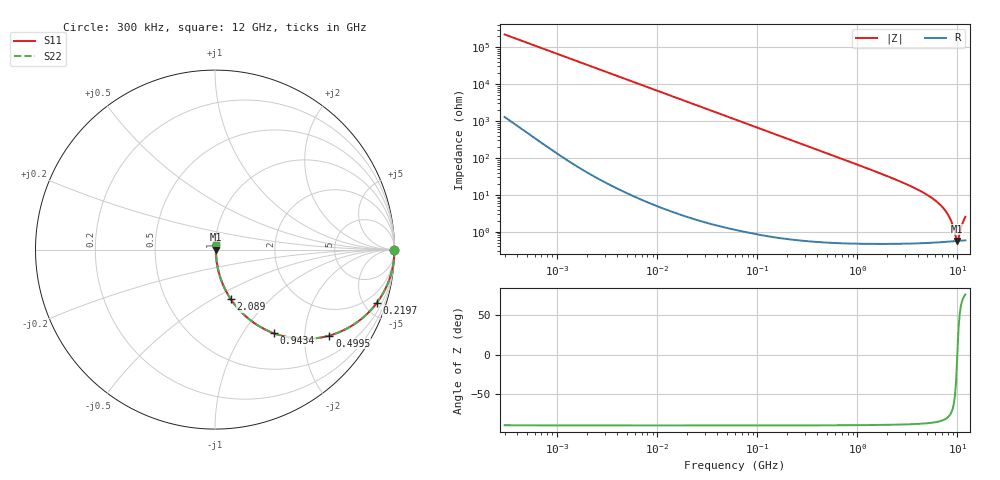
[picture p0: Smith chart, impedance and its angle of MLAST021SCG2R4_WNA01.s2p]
! MLAST021SCG2R4_WNA01  S-PARAMETER MODEL  ( General Type )
! Model Generated by TAIYO YUDEN Corporation (http://www.ty-top.com)
! Version 1.0
! TAIYO YUDEN Control No. 220901
! Copyright(c) 2022 TAIYO YUDEN CO.,LTD. All Rights Reserved.
! Product Description (link to TY-COMPAS)
! https://ds.yuden.co.jp/TYCOMPAS/or/detail?pn=MLAST021SCG2R4BWNA01&u=M
! Products Name : Multilayer Ceramic Capacitors
! Characteristics :
!  Capacitance : 2.4 pF , Rated Voltage : 25V , TCC : CG / C0G
!  Case Size : 0.25 x 0.125 / 0.0098 x 0.0049 [mm/inch] , Thickness : 0.125 / 0.0049 [mm/inch]
!  (Conditions: Temperature = 25 degC , DC Bias Current/Voltage = 0A / 0V)
! External Node Assignments :
!  1  o---| |---o  2
! GND o---------o GND
! Frequency Range : 0.3MHz  -  12000MHz  [ 401 STEP ]
# MHz S RI R 50
! Freq[MHz].  S11 Real  S11 Imag  S21 Real  S21 Imag  S12 Real  S12 Imag  S22 Real  S22 Imag
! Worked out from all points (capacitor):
!   401 points, 300 kHz to 12 GHz, reference 50 ohm
!   read as one part in series: C = 2.4 pF near 316.3 kHz
!   lowest |Z| = 563 mohm at 9.969 GHz (marker M1)
!   series resonance near 9.966 GHz, so ESL is about 110 pH
!   S11 on the Smith chart (normalised r, x): 300 kHz: open; 219.7 MHz: 1.01, -6.05; 499.5 MHz: 1.01, -2.66; 943.4 MHz: 1.01, -1.40; 2.089 GHz: 1.01, -0.61; 12 GHz: 1.01, +0.05
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0.3  1 -0.000452  2.84e-06 0.000452  2.84e-06 0.000452  1 -0.000452
1.769972  1 -0.00267  1.06e-05 0.00267  1.06e-05 0.00267  1 -0.00267
10.44266  0.9997 -0.0157  0.000259 0.0157  0.000259 0.0157  0.9997 -0.0157
60  0.9918 -0.0895  0.00817 0.0895  0.00817 0.0895  0.9918 -0.0895
116.3536  0.9701 -0.1697  0.0299 0.1697  0.0299 0.1697  0.9701 -0.1697
219.7372  0.901 -0.2976  0.099 0.2976  0.099 0.2976  0.901 -0.2976
353.9943  0.7782 -0.414  0.2218 0.414  0.2218 0.414  0.7782 -0.414
499.5319  0.6378 -0.4787  0.3622 0.4787  0.3622 0.4787  0.6378 -0.4787
686.4755  0.482 -0.4972  0.518 0.4972  0.518 0.4972  0.482 -0.4972
943.3804  0.3293 -0.4666  0.6707 0.4666  0.6707 0.4666  0.3293 -0.4666
1403.667  0.18 -0.3791  0.82 0.3791  0.82 0.3791  0.18 -0.3791
2088.533  0.0884 -0.2762  0.9116 0.2762  0.9116 0.2762  0.0884 -0.2762
4158.869  0.0217 -0.1284  0.9783 0.1284  0.9783 0.1284  0.0217 -0.1284
6354.153  0.00888 -0.061  0.9911 0.061  0.9911 0.061  0.00888 -0.061
7254.098  0.00705 -0.0424  0.9929 0.0424  0.9929 0.0424  0.00705 -0.0424
8064.993  0.00614 -0.028  0.9939 0.028  0.9939 0.028  0.00614 -0.028
8732.115  0.00574 -0.0174  0.9943 0.0174  0.9943 0.0174  0.00574 -0.0174
9454.42  0.00558 -0.00691  0.9944 0.00691  0.9944 0.00691  0.00558 -0.00691
9968.853  0.0056 3.8e-05  0.9944 -3.8e-05  0.9944 -3.8e-05  0.0056 3.8e-05
10236.47  0.00564 0.00351  0.9944 -0.00351  0.9944 -0.00351  0.00564 0.00351
11380.75  0.00606 0.0174  0.9939 -0.0174  0.9939 -0.0174  0.00606 0.0174
12000  0.00642 0.0244  0.9936 -0.0244  0.9936 -0.0244  0.00642 0.0244
